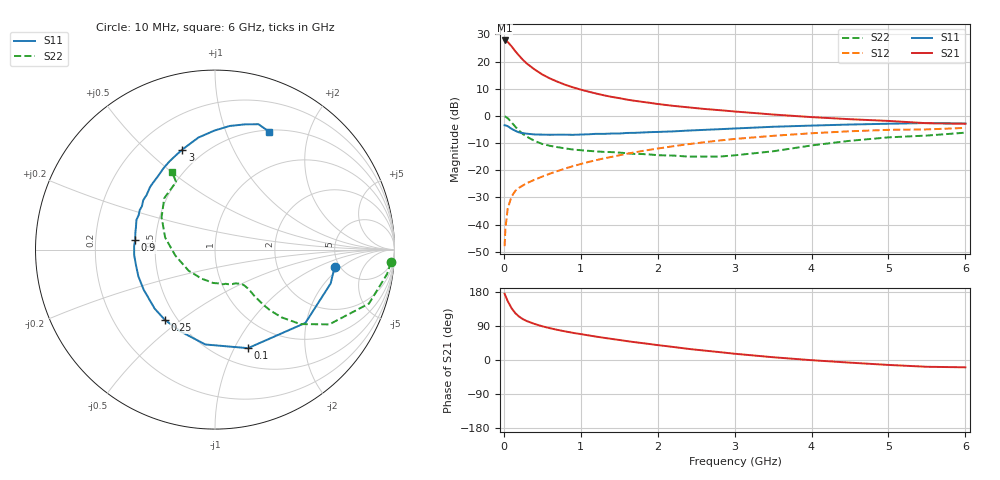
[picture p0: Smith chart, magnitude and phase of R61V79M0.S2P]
! SIEMENS Small Signal Semiconductors
! BFR193
! Si NPN RF Bipolar Junction Transistor in SOT23
! VCE = 1.75 V  IC = 9 mA
! Common Emitter S-Parameters:  May  1996
# GHz  S  MA  R  50
!  f  S11  S21  S12  S22
! GHz  MAG  ANG  MAG  ANG  MAG  ANG  MAG  ANG
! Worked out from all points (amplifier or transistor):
!   36 points, 10 MHz to 6 GHz, reference 50 ohm
!   highest |S21| = 27.8 dB at 10 MHz (marker M1)
!   |S21| within 3 dB of that: start of sweep to 123.2 MHz
!   unconditionally stable (mu >= 1): 742.2 MHz to 2.044 GHz
!   at 250 MHz: K = 0.62, MSG = 23.1 dB, |S12| = -25.5 dB
!   at 1.4 GHz: K = 1.04, MAG = 9.8 dB, |S12| = -15.1 dB
!   at 6 GHz: K = 0.96, MSG = 0.8 dB, |S12| = -4.4 dB
!   S11 on the Smith chart (normalised r, x): 10 MHz: 4.52, -1.61; 100 MHz: 0.69, -1.13; 250 MHz: 0.43, -0.44; 900 MHz: 0.38, +0.05; 3 GHz: 0.38, +0.65; 6 GHz: 0.52, +1.43
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0.01  0.6732 -8.3  24.47 175.0  0.004 85.5  0.9827 -4.1
0.02  0.6715 -16.3  24.13 169.7  0.0083 81.8  0.9683 -8.1
0.05  0.6485 -39.0  22.99 155.6  0.0196 73.9  0.9092 -19.3
0.1  0.5791 -71.5  19.12 136.8  0.0328 61.8  0.7609 -33.2
0.15  0.5313 -95.8  15.46 123.4  0.0419 56.0  0.6315 -41.1
0.2  0.4951 -112.7  12.8 114.2  0.0476 54.2  0.5315 -45.4
0.25  0.4809 -125.6  10.7 107.6  0.0528 53.2  0.4603 -47.7
0.3  0.4702 -135.7  9.169 102.6  0.0579 53.5  0.4134 -48.7
0.4  0.4558 -150.9  7.154 95.1  0.0669 55.5  0.3462 -49.6
0.5  0.4521 -160.9  5.787 89.0  0.0764 57.2  0.3043 -49.6
0.6  0.4488 -169.1  4.883 83.9  0.0865 58.5  0.2814 -49.8
0.7  0.4512 -176.1  4.241 79.4  0.0968 59.7  0.2655 -50.4
0.9  0.4484 173.0  3.345 71.6  0.119 61.0  0.2401 -52.3
1.1  0.4583 163.8  2.798 65.0  0.1419 61.3  0.2276 -56.2
1.3  0.4666 155.7  2.396 58.6  0.1651 60.7  0.2175 -60.4
1.6  0.4854 145.5  1.994 49.8  0.2009 58.9  0.2058 -69.4
2.2  0.5185 127.6  1.532 34.5  0.2761 53.1  0.1862 -93.4
3  0.5864 108.1  1.206 16.5  0.3762 42.3  0.1881 -140.8
3.5  0.6308 98.5  1.06 7.3  0.4299 34.6  0.2231 -171.2
4.5  0.6937 83.2  0.869 -7.0  0.5216 19.3  0.3482 148.7
5.5  0.7394 70.9  0.733 -17.9  0.5643 3.9  0.4347 119.9
6  0.7224 65.2  0.718 -19.3  0.601 -0.6  0.4912 119.0
